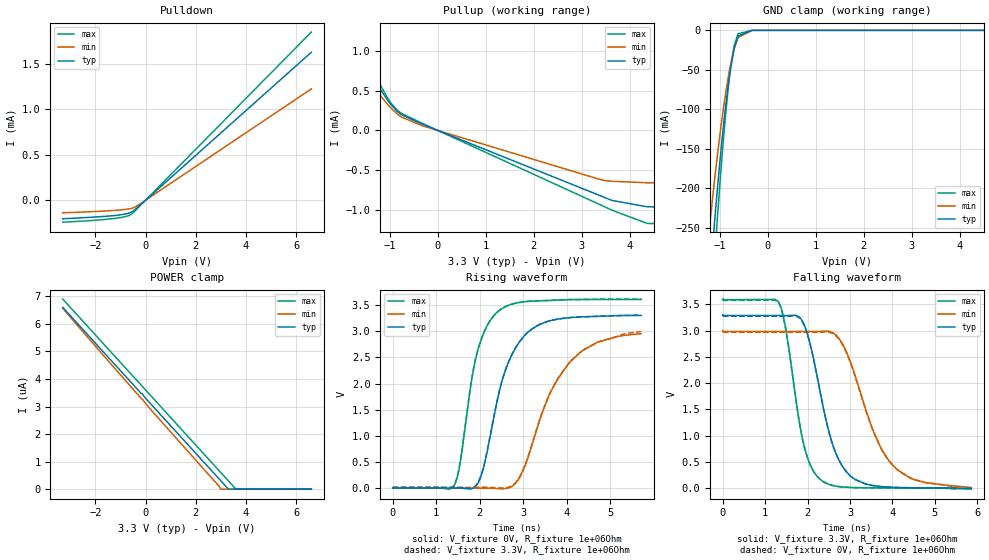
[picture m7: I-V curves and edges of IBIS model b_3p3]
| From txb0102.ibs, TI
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|   b_3p3 Model
[Model]   b_3p3
Model_type   I/O
Polarity   Non-Inverting
Enable   Active-High
Vinl = 1.155
Vinh = 2.145
Vmeas = 1.65
Vref = 0
Cref = 2pF
Rref = 1e6
|   typ   min   max
|   (nom PVT)   (fast PVT)   (slow PVT)
C_comp   1.055e-11   1.055e-11   1.055e-11
[Model spec]
|subparameter
Vinl   1.155   1.05   1.26
Vinh   2.145   1.95   2.34
| Where nom  PVT is Nominal Process, 3.3V, 27C
|   Fast PVT is Strong Process,  3.6V, -40C
|   Slow PVT is Weak Process,   3V, 125C
[Voltage Range]   3.3   3   3.6
|Junction Temperature
[Temperature Range]   27   125   -40
[Pullup Reference]   3.3   3   3.6
[Pulldown Reference]   0   0   0
[Power Clamp Reference]   3.3   3   3.6
[GND Clamp Reference]   0   0   0
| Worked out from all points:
|   slope of the pulldown table from 0 to 0.495 V, typ, clamps not added: 4.06 kohm
|   slope of the pullup table from 0 to 0.495 V, typ, clamps not added: 4.12 kohm
|   falling waveform, V_fixture 3.3V, R_fixture 1e+06Ohm: 20-80 % time 579ps typ, 836ps min, 434ps max; typ from 3.3 V to -0.004 V
|   rising waveform, V_fixture 0V, R_fixture 1e+06Ohm: 20-80 % time 636ps typ, 917ps min, 463ps max; typ from 0 V to 3.3 V
|   rising waveform, V_fixture 3.3V, R_fixture 1e+06Ohm: 20-80 % time 636ps typ, 942ps min, 464ps max; typ from 0.013 V to 3.31 V
|   falling waveform, V_fixture 0V, R_fixture 1e+06Ohm: 20-80 % time 577ps typ, 831ps min, 433ps max; typ from 3.27 V to -0.004 V
[Pulldown]
|   Voltage   I(typ)   I(min)   I(max)
-3.3V     -204.1uA   -138.6uA   -241.6uA
-1.294V   -170.1uA   -113.3uA   -202.3uA
-823.2mV  -152.8uA   -102uA     -181.7uA
-553.2mV  -128.8uA   -89.29uA   -151.4uA
-250.8mV  -61.73uA   -46.35uA   -70.14uA
6.6V      1.624mA    1.221mA    1.845mA
[GND Clamp]
|   Voltage   I(typ)   I(min)   I(max)
-3.3V     -2.598A    -2.054A    -3.033A
-1.255V   -355.5mA   -273.7mA   -430.7mA
-1.195V   -306.7mA   -237.2mA   -370.1mA
-1.109V   -241.5mA   -188.6mA   -288.8mA
-1.053V   -201.7mA   -159mA     -239mA
-920.7mV  -118.4mA   -96.79mA   -134.4mA
-825mV    -68.86mA   -59.22mA   -72.89mA
-774mV    -47.1mA    -42.4mA    -46.7mA
-706.2mV  -24.38mA   -24.28mA   -20.93mA
-618mV    -7.095mA   -9.021mA   -4.295mA
-330mV    -8.359uA   -53.41uA   -585.5nA
6.6V      0A         0A         0A
[Pullup]
|   Voltage   I(typ)   I(min)   I(max)
-3.3V     5.039mA    3.81mA     7.973mA
-1.899V   1.512mA    1.427mA    1.794mA
-1.759V   1.259mA    1.134mA    1.5mA
-1.615V   1.035mA    891.4uA    1.222mA
-1.406V   752.6uA    632.8uA    865.4uA
-1.18V    500.6uA    426.1uA    551.9uA
-972mV    321.4uA    278.9uA    340.3uA
-759mV    198.2uA    168.3uA    214.5uA
-330mV    80.09uA    60.31uA    91.26uA
3.393V    -823.8uA   -618uA     -938.3uA
4.357V    -960.4uA   -658.6uA   -1.17mA
6.6V      -993uA     -678.9uA   -1.223mA
[POWER Clamp]
|   Voltage   I(typ)   I(min)   I(max)
-3.3V     6.601uA    6.565uA    6.901uA
-207.6mV  3.508uA    3.327uA    3.81uA
-122.1mV  3.452uA    3.251uA    3.722uA
63mV      3.237uA    3.04uA     3.537uA
2.851V    448.9nA    182.1nA    748.8nA
2.997V    303.1nA    0A         603nA
3.303V    0A         0A         296.7nA
3.598V    0A         0A         0A
6.6V      0A         0A         0A
[Ramp]
R_load = 1e+06
|   typ   min   max
dV/dt_r   1.96989/6.26011e-10   1.78606/9.30193e-10   2.15109/4.52684e-10
dV/dt_f   1.97147/5.73696e-10   1.79081/8.35363e-10   2.15083/4.25194e-10
[Falling Waveform]
V_fixture = 3.3V
V_fixture_min = 3V
V_fixture_max = 3.6V
R_fixture = 1e+06Ohm
|   Time   V(typ)   V(min)   V(max)
0s        3.3V       3V         3.6V
1.314ns   3.286V     2.983V     3.549V
1.476ns   3.285V     2.983V     3.084V
1.884ns   3.172V     2.983V     926mV
2.31ns    1.78V      2.985V     156.1mV
2.66ns    678.1mV    2.922V     38.26mV
3.124ns   162.9mV    2.136V     8.289mV
3.538ns   47.84mV    1.111V     4.04mV
4.01ns    14.27mV    433.8mV    2.219mV
5.86ns    -3.927mV   10.13mV    -20.61mV
[Rising Waveform]
V_fixture = 0V
V_fixture_min = 0V
V_fixture_max = 0V
R_fixture = 1e+06Ohm
|   Time   V(typ)   V(min)   V(max)
0s        88.29nV    19.79uV    51.36nV
1.396ns   784.7uV    -13.4uV    25.8mV
1.544ns   43.71uV    -3.415uV   455.4mV
1.824ns   -8.177mV   245uV      2.123V
1.964ns   102.8mV    601uV      2.663V
2.452ns   1.861V     -10.62mV   3.401V
3.034ns   2.921V     414.4mV    3.564V
3.578ns   3.193V     1.748V     3.588V
4.1ns     3.263V     2.436V     3.606V
5.712ns   3.302V     2.954V     3.608V
[Rising Waveform]
V_fixture = 3.3V
V_fixture_min = 3V
V_fixture_max = 3.6V
R_fixture = 1e+06Ohm
|   Time   V(typ)   V(min)   V(max)
0s        13.3mV     15.98mV    12.78mV
1.396ns   14.08mV    15.95mV    38.59mV
1.544ns   13.34mV    15.96mV    467.9mV
1.824ns   5.197mV    16.21mV    2.132V
1.964ns   116.2mV    16.56mV    2.672V
2.452ns   1.871V     5.406mV    3.402V
3.034ns   2.925V     430.6mV    3.565V
3.576ns   3.194V     1.754V     3.588V
4.096ns   3.263V     2.438V     3.606V
5.708ns   3.307V     2.994V     3.616V
[Falling Waveform]
V_fixture = 0V
V_fixture_min = 0V
V_fixture_max = 0V
R_fixture = 1e+06Ohm
|   Time   V(typ)   V(min)   V(max)
0s        3.273V     2.967V     3.574V
1.314ns   3.273V     2.967V     3.536V
1.476ns   3.272V     2.967V     3.071V
1.884ns   3.158V     2.967V     919.5mV
2.308ns   1.776V     2.969V     156.3mV
2.66ns    673mV      2.906V     37.95mV
3.08ns    184.9mV    2.228V     9.189mV
3.536ns   47.47mV    1.105V     3.964mV
4.01ns    13.89mV    429mV      2.126mV
5.568ns   -4.08mV    9.915mV    -21.07mV
